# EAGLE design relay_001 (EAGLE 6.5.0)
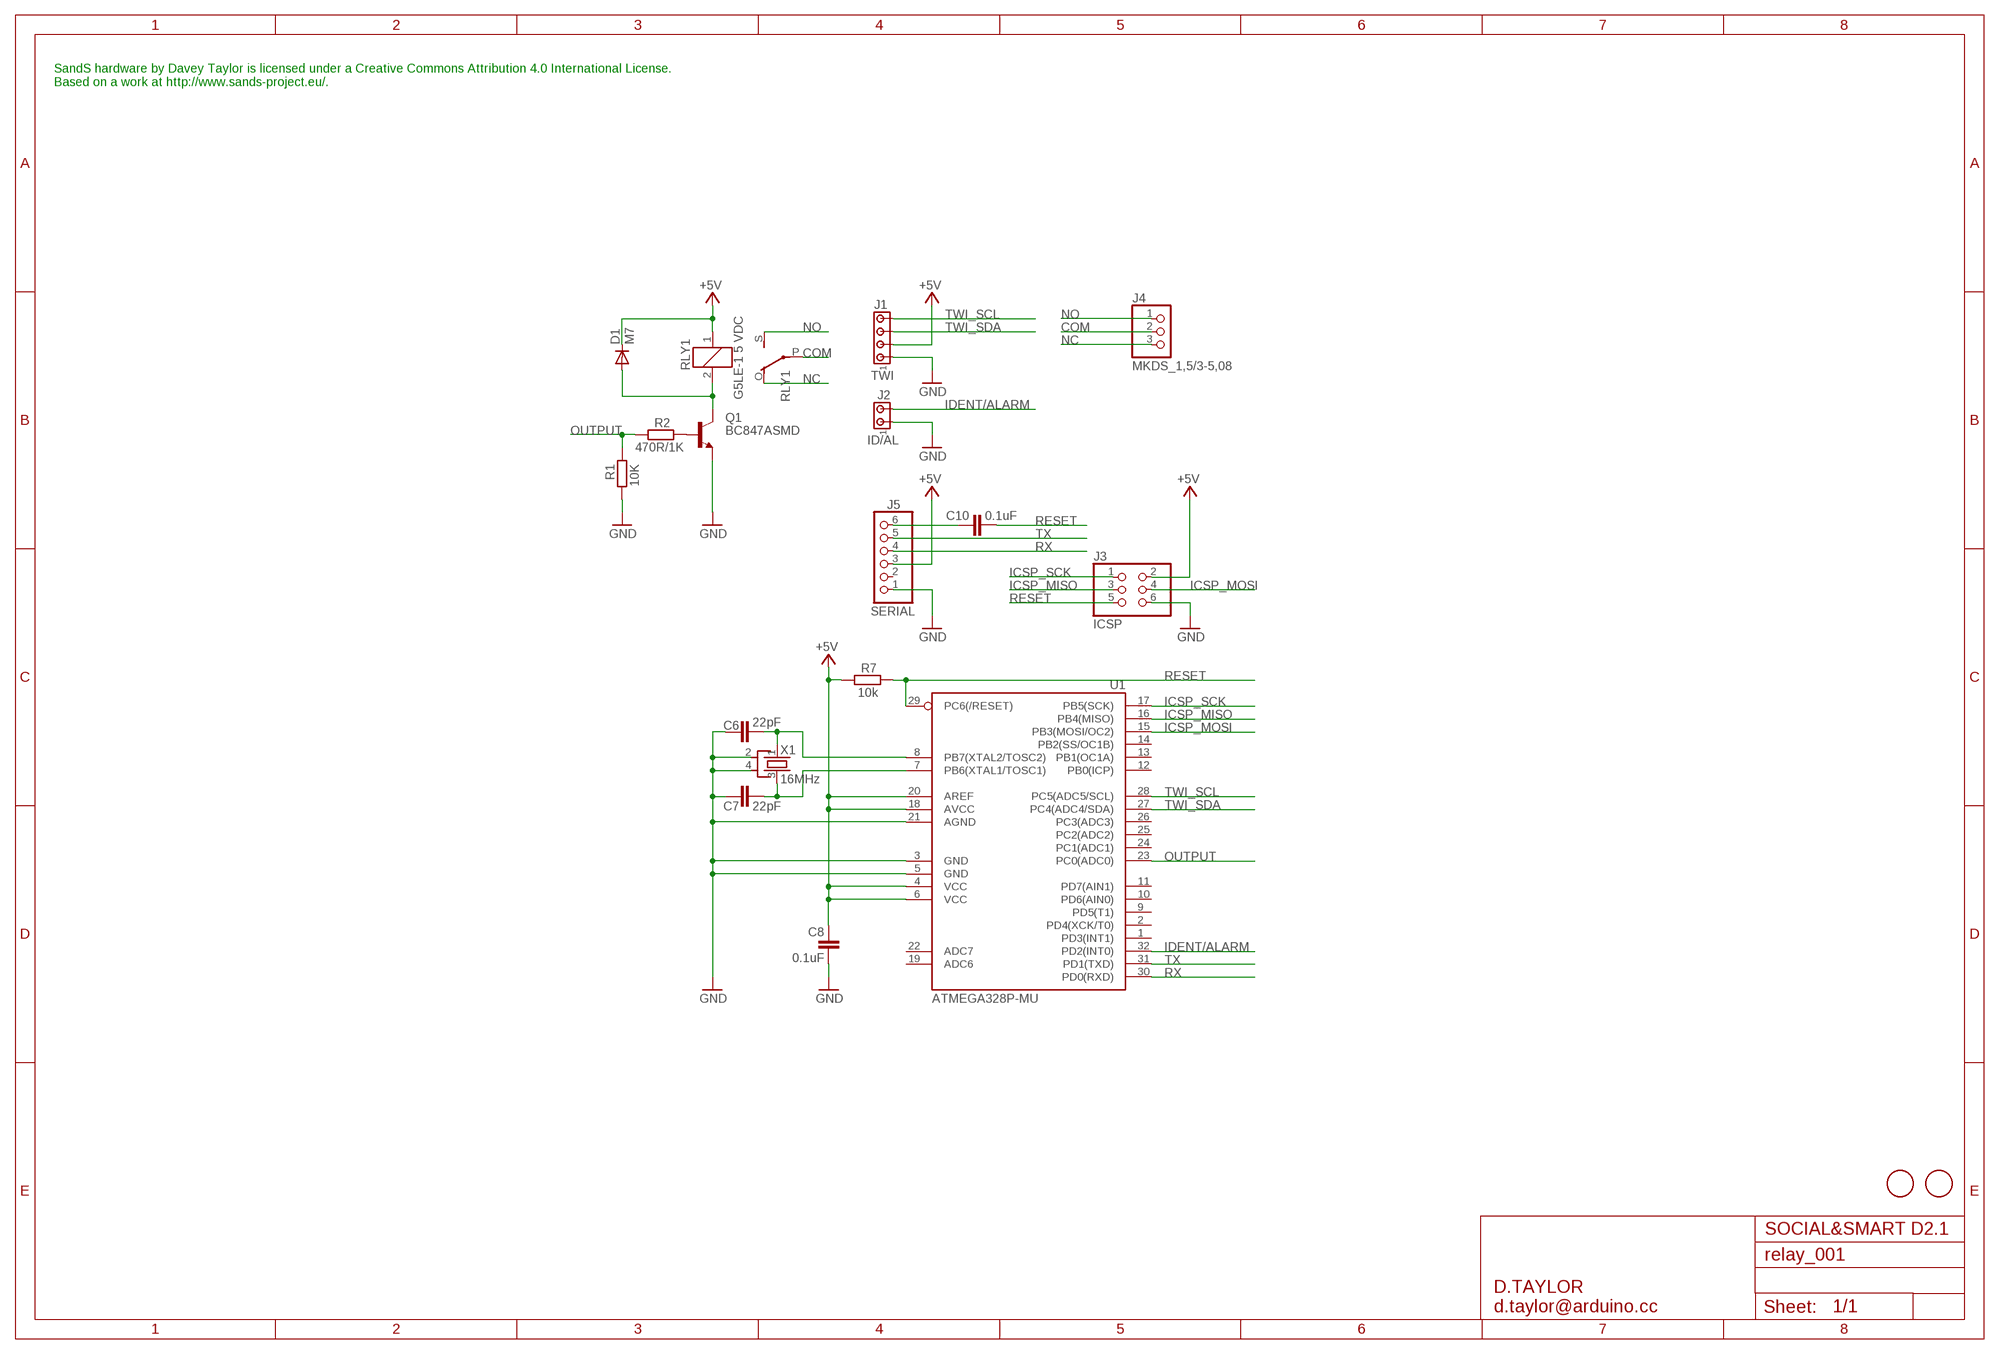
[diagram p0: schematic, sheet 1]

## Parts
C6  22pF  C-EUC0603  [C0603]
C7  22pF  C-EUC0603  [C0603]
C8  0.1uF  C-EUC0603  [C0603]
C10  0.1uF  C-EUC0603  [C0603]
D1  M7  DIODE_DIODE-SMB  [DIODE_SMB]
J1  TWI  MTA04-100  [10X04MTA]
J2  ID/AL  MTA02-100  [10X02MTA]
J3  ICSP  PINHD-2X3  [2X03]
J4  MKDS_1,5/3-5,08  [MKDS1,5/3-5,08]
J5  SERIAL  PINHD-1X6  [1X06]
Q1  BC847ASMD  [SOT23]
R1  10K  R-EU_R0603  [R0603]
R2  470R/1K  R-EU_R0603  [R0603]
R7  10k  R-EU_R0603  [R0603]
RLY1  G5LE-1 5 VDC  G5LE  [G5LE]
U1  ATMEGA328P-MU  [MLF32-M1-A]
U$5  FIDUCIALMOUNT  [FIDUCIA-MOUNT]
U$6  FIDUCIALMOUNT  [FIDUCIA-MOUNT]
X1  16MHz  CRYSTAL-KX7  [XTAL-3.2-2.5]

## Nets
+5V: C8.1 D1.C J1.2 J3.2 J5.3 R7.1 RLY1.1 U1.4(VCC) U1.6(VCC) U1.18(AVCC) U1.20(AREF)
COM: J4.2 RLY1.P(2:P)
GND: C6.1 C7.1 C8.2 J1.1 J2.1 J3.6 J5.1 Q1.2(E) R1.2 U1.3(GND) U1.5(GND) U1.21(AGND) X1.2(SH1) X1.4(SH2)
ICSP_MISO: J3.3 U1.16(PB4(MISO))
ICSP_MOSI: J3.4 U1.15(PB3(MOSI/OC2))
ICSP_SCK: J3.1 U1.17(PB5(SCK))
IDENT/ALARM: J2.2 U1.32(PD2(INT0))
N$2: D1.A Q1.3(C) RLY1.2
N$4: Q1.1(B) R2.1
N$6: C6.2 U1.8(PB7(XTAL2/TOSC2)) X1.1(X1)
N$7: C7.2 U1.7(PB6(XTAL1/TOSC1)) X1.3(X2)
N$9: C10.1 J5.6
NC: J4.3 RLY1.O(2:O)
NO: J4.1 RLY1.S(2:S)
OUTPUT: R1.1 R2.2 U1.23(PC0(ADC0))
RESET: C10.2 J3.5 R7.2 U1.29(PC6(/RESET))
RX: J5.4 U1.30(PD0(RXD))
TWI_SCL: J1.4 U1.28(PC5(ADC5/SCL))
TWI_SDA: J1.3 U1.27(PC4(ADC4/SDA))
TX: J5.5 U1.31(PD1(TXD))
Unconnected: J5.2 U1.1(PD3(INT1)) U1.2(PD4(XCK/T0)) U1.9(PD5(T1)) U1.10(PD6(AIN0)) U1.11(PD7(AIN1)) U1.12(PB0(ICP)) U1.13(PB1(OC1A)) U1.14(PB2(SS/OC1B)) U1.19(ADC6) U1.22(ADC7) U1.24(PC1(ADC1)) U1.25(PC2(ADC2)) U1.26(PC3(ADC3))

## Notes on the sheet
- SandS hardware by Davey Taylor is licensed under a Creative Commons Attribution 4.0 International License.
  Based on a work at http://www.sands-project.eu/.
- SOCIAL&SMART D2.1
- D.TAYLOR
  d.taylor@arduino.cc

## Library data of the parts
C6-C8 C10 = rcl:C-EU: CAPACITOR, European symbol
D1 = stickduino:DIODE_DIODE-: DIODE
J1 = con-amp:MTA04-100: AMP connector
J2 = con-amp:MTA02-100: AMP connector
J3 = pinhead:PINHD-2X3: PIN HEADER
J4 = d_taylor:MKDS_1,5/3-5,08: MKDSN 1,5/ 3-5,08 Printklemme Nennstrom: 13,5 A Nennspannung: 250 V Rastermaß: 5,08 mm Polzahl: 3 Anschlussart: Schraubanschluss Montage: Löten Anschlussrichtung Leiter/Platine: 0 ° Artikelnummer: 1729131 Source: http://eshop.phoenixcontact.com .. 1729131.pdf; MPN: SMKDSN1,5/3-5,08; OC_FARNELL: 1792904; OC_NEWARK: 70R0299
J5 = pinhead:PINHD-1X6: PIN HEADER
Q1 = transistor-npn:BC847*: NPN Transistor
R1 R2 = SmartPrj:R-EU_: RESISTOR, European symbol
R7 = rcl:R-EU_: RESISTOR, European symbol
RLY1 = relay:G5LE: RELAY 1 x switch, 10 A/120 V AC, 8 A/30 V DC, Omron; OC_FARNELL: unknown; OC_NEWARK: unknown
U1 = d_taylor:ATMEGA*: MICROCONTROLLER 8 Kbytes FLASH 1 kbytes SRAM 512 bytes EEPROM USART 6-channel 10 bit ADC 2-channel 8 bit ADC Source: avr.lbr
U$5 U$6 = SmartPrj:FIDUCIALMOUNT
X1 = d_taylor:CRYSTAL-KX7

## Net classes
1 PWR: width 0.406 mm, clearance 0.254 mm

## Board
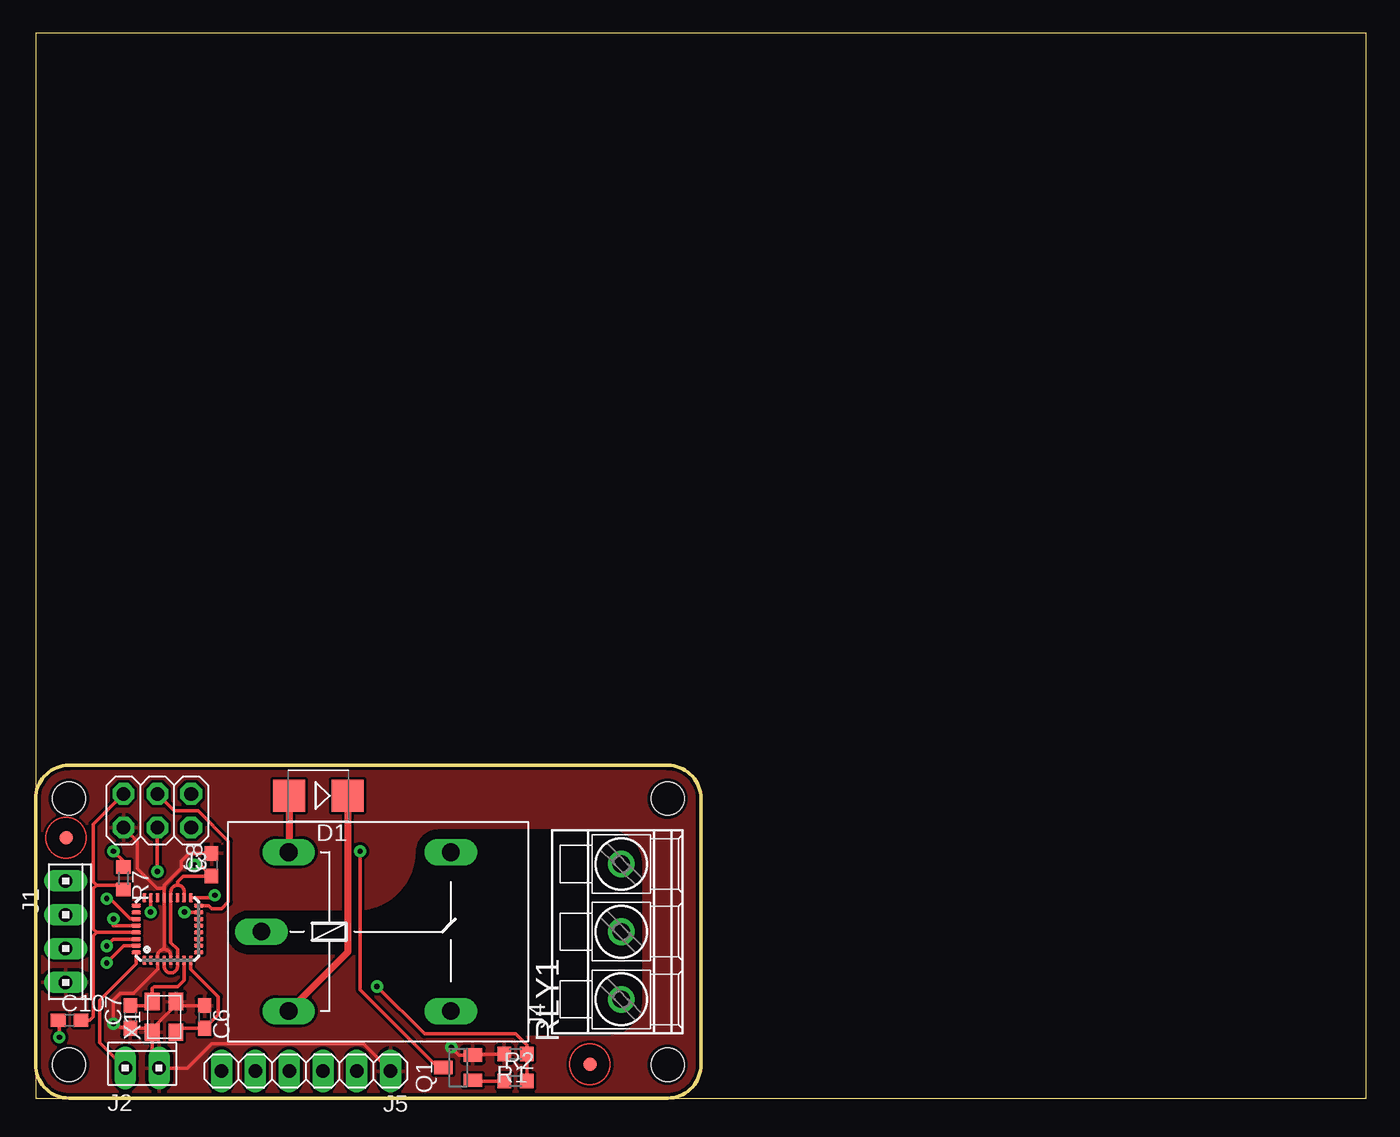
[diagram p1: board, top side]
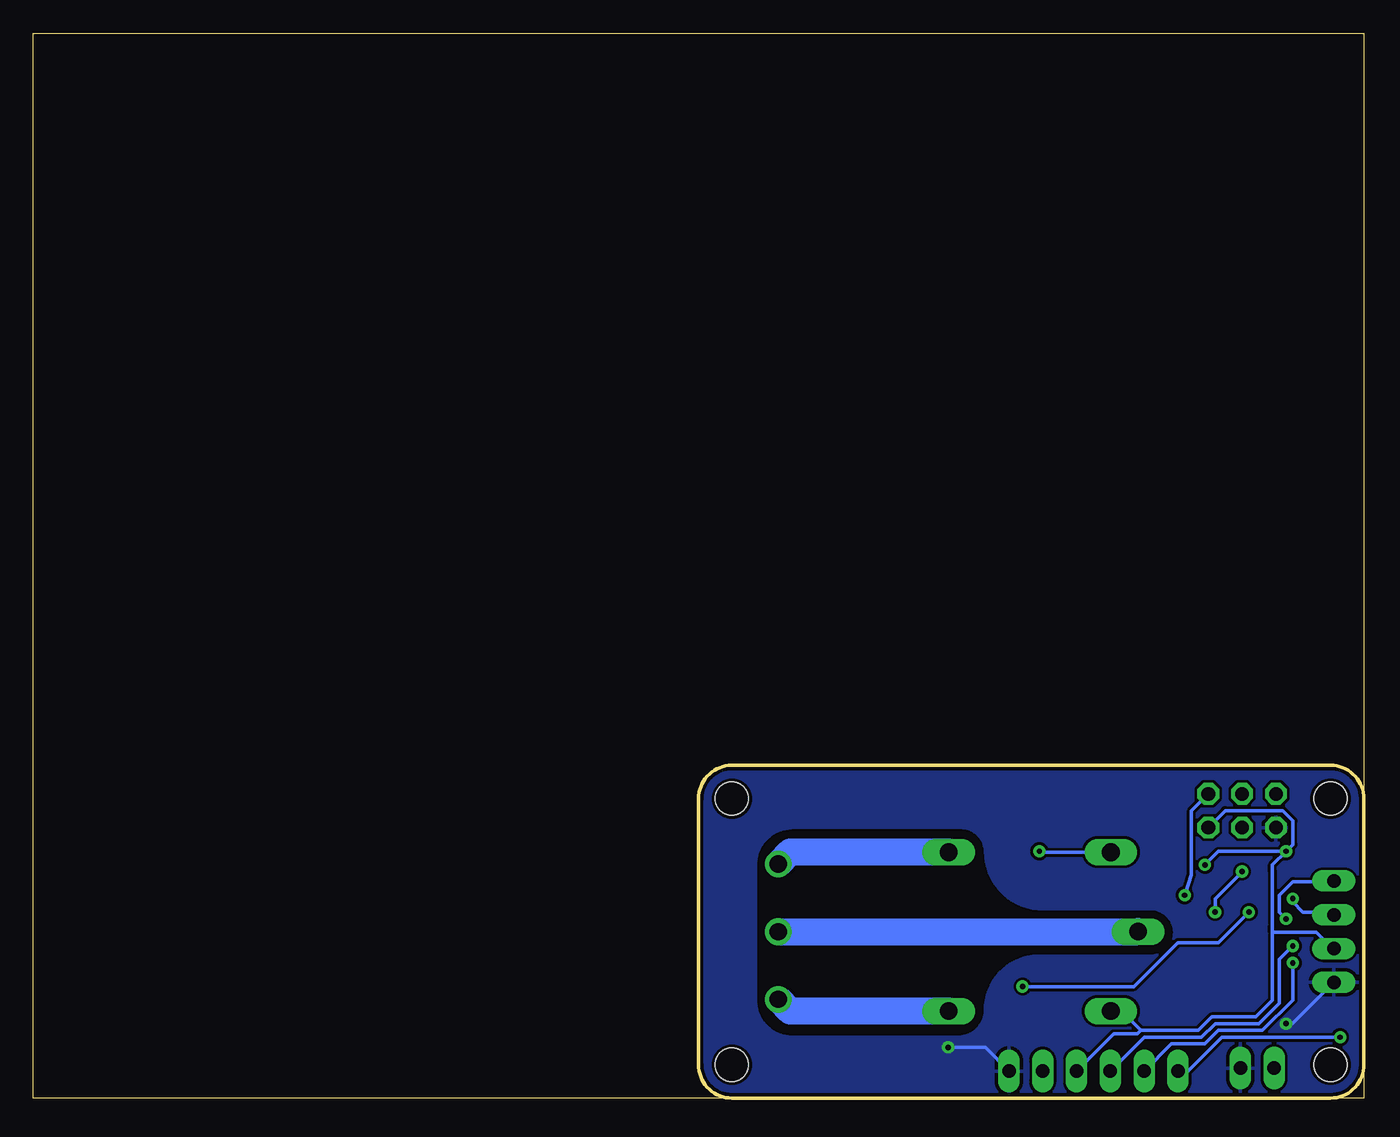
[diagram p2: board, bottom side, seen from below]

Size 100 x 80 mm. Coordinates in mm from the lower left corner, seen from the top.
Outline: 0,0 100,0 100,80 0,80 0,0
Outline: 2.5,0 47.5,0 arc90 50,2.5 50,22.5 arc90 47.5,25 2.5,25 arc90 0,22.5 0,2.5 arc90 2.5,0
Copper layers (1*16): Top 0.035mm / dielectric 1.5mm / Bottom 0.035mm
Design rules "smartprj-mini *": minimum track width 8mil, minimum drill 16mil, track to track 8mil, track to pad 8mil, pad to pad 0.200659375mm, via to via 8mil, smd to smd 4mil, copper to edge 10mil, drill to drill 8mil, minimum pad ring 12mil, minimum via ring 10mil, stop-mask expansion 2mil, vias tented up to drill 20mil, thermal gap 10mil
Holes 2.5 mm at 2.5,22.5 2.5,2.5 47.5,2.5 47.5,22.5
tRestrict: area 14.5,4.8 to 45.5,20.1
bRestrict: area 14.5,4.8 to 45.5,20.1

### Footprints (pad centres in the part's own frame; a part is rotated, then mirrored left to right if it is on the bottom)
C0603 = smd 1.1 x 1: 1 -0.85,0; 2 0.85,0
DIODE_SMB = smd 2.4 x 2.4: A 2.2,0; C -2.2,0
10X04MTA = drill 1.016 long: 1 3.81,0; 2 1.27,0; 3 -1.27,0; 4 -3.81,0
10X02MTA = drill 1.016 long: 1 1.27,0; 2 -1.27,0
2X03 = drill 1.016 octagon: 1 -2.54,-1.27; 2 -2.54,1.27; 3 0,-1.27; 4 0,1.27; 5 2.54,-1.27; 6 2.54,1.27
MKDS1,5/3-5,08 = drill 1.3 pad 2: 1 -5.08,0; 2 0,0; 3 5.08,0
1X06 = drill 1.016 long: 1 -6.35,0; 2 -3.81,0; 3 -1.27,0; 4 1.27,0; 5 3.81,0; 6 6.35,0
SOT23 = smd 1 x 1.4: 1 -0.95,-1.1; 2 0.95,-1.1; 3 0,1.1
R0603 = smd 1 x 1.1: 1 -0.85,0; 2 0.85,0
G5LE = drill 1.321 long: 1 -7.493,-5.969; 2 -7.493,5.969; O 4.699,5.969; P -9.525,0; S 4.699,-5.969
MLF32-M1-A = smd 0.7 x 0.3: 1 -2.35,1.75; 2 -2.35,1.25; 3 -2.35,0.75; 4 -2.35,0.25; 5 -2.35,-0.25; 6 -2.35,-0.75; 7 -2.35,-1.25; 8 -2.35,-1.75; 17 2.35,-1.75; 18 2.35,-1.25; 19 2.35,-0.75; 20 2.35,-0.25; 21 2.35,0.25; 22 2.35,0.75; 23 2.35,1.25; 24 2.35,1.75 | smd 0.3 x 0.7: 9 -1.75,-2.35; 10 -1.25,-2.35; 11 -0.75,-2.35; 12 -0.25,-2.35; 13 0.25,-2.35; 14 0.75,-2.35; 15 1.25,-2.35; 16 1.75,-2.35; 25 1.75,2.35; 26 1.25,2.35; 27 0.75,2.35; 28 0.25,2.35; 29 -0.25,2.35; 30 -0.75,2.35; 31 -1.25,2.35; 32 -1.75,2.35
FIDUCIA-MOUNT = smd 1.016 x 1.016: P$1 0,0
XTAL-3.2-2.5 = smd 1.3 x 1.1: 1 -1.15,-0.9; 2 1.15,-0.9; 3 1.15,0.9; 4 -1.15,0.9

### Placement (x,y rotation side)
C6  12.7,6.1 270 top
C7  7.11,6.1 90 top
C8  13.21,17.53 90 top
C10  2.54,5.84 0 top
D1  21.24,22.72 180 top
J1  2.25,12.5 270 top
J2  8,2.25 0 top
J3  9.14,21.59 180 top
J4  44,12.5 90 top
J5  20.32,2.03 180 top
Q1  31.75,2.29 90 top
R1  36.07,3.3 180 top
R2  36.07,1.27 0 top
R7  6.6,16.51 270 top
RLY1  26.5,12.5 0 top
U1  9.91,12.7 90 top
U$5  2.29,19.56 0 top
U$6  41.66,2.54 0 top
X1  9.65,6.1 90 top

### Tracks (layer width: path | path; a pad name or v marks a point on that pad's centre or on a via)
+5V  (via drill 0.41)
  Top 0.254: 11.18,15.32 U1.18 | 11.18,15.05 U1.18 | R7.1 6.6,17.78 v5.84,18.54 | U1.4 9.66,9.9 arc90 10.16,9.4 arc90 10.66,9.89 U1.6 10.67,10.36 10.67,11.18 10.16,11.69 U1.20 10.16,15.49 arc-90 10.67,16 | U1.18 11.16,15.51 arc90 10.67,16 | 10.67,16 10.67,16.26 11.09,16.68 C8.1 12.36,17.53 v11.94,17.53
  Top 0.508: D1.C 23.44,10.97 RLY1.1
  Bottom 0.254: J5.3 18.8,4.83 17.02,4.83 16.76,5.08 | 16.76,5.08 12.45,5.08 11.43,6.1 8.13,6.1 7.37,6.86 6.86,7.37 6.86,8.89 6.86,9.14 6.86,12.45 | 6.86,12.95 6.86,15.75 6.86,17.02 6.86,17.53 v5.84,18.54 | 6.86,12.95 6.86,12.45 | 6.86,12.45 3.56,12.45 2.51,11.43 J1.2 | 6.86,12.45 6.86,12.95 | 6.86,12.95 6.86,12.45 | J3.2 10.41,21.59 6.1,21.59 5.33,20.83 5.33,19.05 v5.84,18.54 | RLY1.1 18.21,6.53 16.76,5.08 | v11.94,17.53 10.92,18.54 v5.84,18.54
COM
  Bottom 2.032: J4.2 RLY1.P
GND  (via drill 0.41)
  Top 0.254: 10.16,10.16 U1.5 10.16,10.68 arc90 9.66,11.18 | 9.14,10.35 U1.3 | 9.65,11.18 9.66,11.18 | 9.66,11.18 9.66,11.18 arc-90 9.65,11.18 | 9.65,11.18 U1.21 | 9.14,10.35 U1.3 | U1.21 | 9.14,10.35 9.14,10.66 arc-90 9.66,11.18 | X1.4 8.45,5.25 C7.1 7.02,5.33 6.35,5.33 v5.84,5.59 5.84,7.37 6.35,7.87 7.37,7.87 7.62,8.13 9.16,9.66 U1.3 | C6.1 10.85,6.95 X1.2 10.55,7 9.65,6.1 8.75,5.2 X1.4 | U1.21 9.66,15.74 9.65,15.75 | 9.65,15.75 9.14,15.75 7.62,17.27 7.62,19.3 J3.6 | X1.4 8.75,2.77 J2.1 11.4,2.25 13.21,4.06 24.64,4.06 J5.1 | 9.65,15.75 9.65,16 10.92,17.27 10.92,17.78 11.52,18.38 C8.2 | R1.2 32.92,3.3 Q1.2 31.82,3.24 v31.24,3.81
  Bottom 0.254: v5.84,5.59 5.36,5.59 J1.1 | v31.24,3.81 28.45,3.81 J5.1
  pour Top: 0.5,22.5 arc-90 2.5,24.5 47.5,24.5 arc-90 49.5,22.5 49.5,2.5 arc-90 47.5,0.5 2.5,0.5 arc-90 0.5,2.5
  pour Bottom: 0.5,22.5 arc-90 2.5,24.5 47.5,24.5 arc-90 49.5,22.5 49.5,2.5 arc-90 47.5,0.5 2.5,0.5 arc-90 0.5,2.5
ICSP_MISO
  Top 0.254: U1.16 12.98,14.45 13.21,14.22 13.72,14.22 13.97,14.22 14.48,14.73 14.48,19.3 12.19,21.59 10.41,21.59 J3.3
ICSP_MOSI  (via drill 0.41)
  Top 0.254: J3.4 v9.14,17.02 | U1.15 11.2,13.95 v11.18,13.97
  Bottom 0.254: v9.14,17.02 11.18,14.99 v11.18,13.97
ICSP_SCK  (via drill 0.41)
  Top 0.254: U1.17 13.27,15.05 v13.46,15.24
  Bottom 0.254: v13.46,15.24 12.95,16.76 12.95,19.81 12.95,21.59 J3.1
IDENT/ALARM
  Top 0.254: J2.2 4.83,4.16 4.83,7.37 7.56,10.1 U1.32
N$2  (via drill 0.41)
  Top 0.254: Q1.3 30.23,2.29 24.38,8.13 v24.38,18.54
  Top 0.508: D1.A 19.04,18.51 RLY1.2
  Bottom 0.254: v24.38,18.54 24.31,18.47 RLY1.2
N$4
  Top 0.254: R2.1 32.92,1.27 Q1.1
N$6
  Top 0.254: X1.1 10.85,5.25 C6.2 13.72,6.26 13.72,7.62 11.66,9.68 U1.8
N$7
  Top 0.254: C7.2 8.45,6.95 X1.3 8.75,8.24 8.89,8.38 10.41,8.38 10.67,8.38 11.16,8.87 U1.7
N$9  (via drill 0.41)
  Top 0.254: v1.78,4.57 1.78,5.84 C10.1
  Bottom 0.254: J5.6 13.21,2.03 10.67,4.57 v1.78,4.57
NC
  Bottom 2.032: RLY1.O 43.11,18.47 J4.3
NO
  Bottom 2.032: RLY1.S 43.11,6.53 J4.1
OUTPUT  (via drill 0.41)
  Top 0.254: R2.2 R1.1 36.92,3.98 36.07,4.83 29.21,4.83 v25.65,8.38 | U1.23 8.66,13.99 v8.64,13.97
  Bottom 0.254: v25.65,8.38 17.27,8.38 13.97,11.68 10.92,11.68 v8.64,13.97
RESET
  Top 0.254: U1.29 5.84,12.45 4.57,12.45 | 4.57,12.45 4.32,12.7 4.32,15.75 4.57,16 | 4.57,16 4.32,16.26 4.32,20.57 J3.5 | C10.2 4.06,5.84 4.32,6.1 4.32,12.19 4.57,12.45 | R7.2 6.6,16 4.57,16
RX  (via drill 0.41)
  Top 0.254: U1.30 7.56,11.94 5.84,11.94 v5.33,11.43
  Bottom 0.254: v5.33,11.43 6.35,10.41 6.35,7.11 6.86,6.6 7.87,5.59 11.18,5.59 12.19,4.57 16.51,4.57 J5.4
TWI_SCL  (via drill 0.41)
  Top 0.254: U1.28 5.84,12.95 v5.84,13.46
  Bottom 0.254: v5.84,13.46 6.35,13.97 6.35,15.24 5.33,16.26 2.29,16.26 2.29,16.31 J1.4
TWI_SDA  (via drill 0.41)
  Top 0.254: v5.33,14.99 5.59,14.99 7.11,13.46 7.56,13.46 U1.27
  Bottom 0.254: J1.3 2.51,13.97 4.57,13.97 5.33,14.73 v5.33,14.99
TX  (via drill 0.41)
  Top 0.254: U1.31 6.6,11.45 v5.33,10.16
  Bottom 0.254: v5.33,10.16 5.33,7.37 7.62,5.08 10.92,5.08 11.94,4.06 14.48,4.06 J5.5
